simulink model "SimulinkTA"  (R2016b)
settings: Solver=VariableStepAuto  StartTime=0.0  StopTime=10000  RelTol=1e-3
libraries: simulink x15, sldrtlib x1
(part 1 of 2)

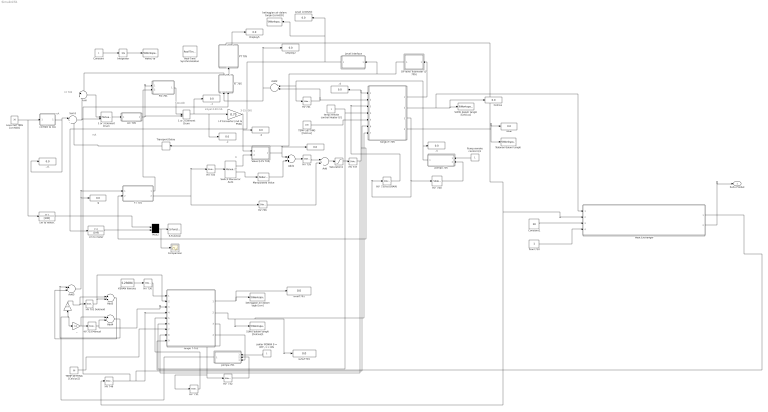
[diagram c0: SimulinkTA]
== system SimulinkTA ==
  note: Cascade
  note: 3-15 PSIG
  note: sinyal 4-20 mA
  note: mA
  note: mA
  note: A
  note: M
  note: LY 705
  ,. : Gain  RequirementInfo={} %GIDa_f98b540b_1780_41dd_a70e_1bad47bc10c1  Gain=1/2
  .{,1..5,9,11} (8 alike) : Display
  .. : Gain  RequirementInfo={} %GIDa_8e0160ac_725a_48f6_95bf_1d56de90cc87  Gain=1/2
  1 or 2 Element Drum : ManualSwitch  RequirementInfo={} %GIDa_50f61c56_16a2_43dc_89b1_2e4d65b653a3  CurrentSetting=0
  1 or 3 Element Drum : ManualSwitch  RequirementInfo={} %GIDa_52ca6b7f_6063_4425_9fdd_553e1b81c659  CurrentSetting=0
  Add : Sum  RequirementInfo={} %GIDa_33aeec0d_9e6c_469e_a3ee_407601759ac2
  Add1 : Sum  RequirementInfo={} %GIDa_8e166b0c_1a9c_4ce2_9319_8c6bd7aad9d2
  Add2 : Sum  RequirementInfo={} %GIDa_713da8c0_9236_4d12_ba44_68ec175b8b10  Inputs=+-
  Add3 : Sum  RequirementInfo={} %GIDa_be23a2ac_e2a6_474d_b9c0_3f98fa9e31fd  Inputs=+-
  Add4 : Sum  RequirementInfo={} %GIDa_40610020_3c23_44b6_97d5_d48497f2e700  Inputs=+-
  Add5 : Sum  RequirementInfo={} %GIDa_806e11a4_cf6f_4655_9173_03499af1af91
  Celcius : Display
  Comparison : Scope
  Constant : Constant  RequirementInfo={} %GIDa_2e5088a9_5b13_476f_95c2_5b910ea94592
  Constant1 : Constant  Value=28
  DP level Trasmitter (LT 705) : Subsystem  RequirementInfo={} %GIDa_91b3a82a_3a49_4232_a21b_3a53aa669424
  Display2 : Display
  Display5 : Display
  FIC 701 : Subsystem  RequirementInfo={} %GIDa_a8cdff3a_9de8_4317_845b_7d10f14f6ae7
  FT 701 : Subsystem  RequirementInfo={} %GIDa_7c1594a4_5410_4ceb_b93e_be43770988d4
  FT 705 : Subsystem  RequirementInfo={} %GIDa_b73ffb92_9bd8_4e1a_9659_5756a25f0d2c
  "HV  731 " : simulink/Math Operations/Slider Gain  low=0  gain=0  high=1
  HV  732 : simulink/Math Operations/Slider Gain  low=0  gain=0  high=1
  "HV  739 to DRAIN " : simulink/Math Operations/Slider Gain  low=0  gain=0  high=1
  "HV  740 " : simulink/Math Operations/Slider Gain  low=0  gain=0  high=1
  HV 701 Selenoid : simulink/Math Operations/Slider Gain  low=0  gain=0  high=1
  HV 730 : simulink/Math Operations/Slider Gain  low=0  gain=0  high=1
  HV 733 Manual : simulink/Math Operations/Slider Gain  low=0  gain=0  high=1
  "HV 734 " : simulink/Math Operations/Slider Gain  low=0  gain=1  high=1
  HV 735 : simulink/Math Operations/Slider Gain  low=0  gain=1  high=1
  "HV 736 " : simulink/Math Operations/Slider Gain  low=0  gain=0  high=1
  "HV 737 " : simulink/Math Operations/Slider Gain  low=0  gain=1  high=1
  "HV 741 " : simulink/Math Operations/Slider Gain  low=0  gain=0  high=1
  HV 746 : simulink/Math Operations/Slider Gain  low=0  gain=0  high=1
  Heat Exchanger : Subsystem
  I-P Converter (mA to PSIG) : Gain  RequirementInfo={} %GIDa_f426d195_d862_463c_9f94_379edd20df78  Gain=0.75
  Integrator : Integrator  RequirementInfo={} %GIDa_73503aa6_2a92_4f4f_9bc4_a531c9719bd6
  KERAN liter/sec : Constant  RequirementInfo={} %GIDa_919a1f09_4405_4c75_a137_f373f18aebd0  Value=0.23084
  LIC 705 : Subsystem  RequirementInfo={} %GIDa_369aca42_e7c0_40f4_8e28_9a6ab2f6df2e
  Level (cmH2O) : Display
  Level SETTING [cmH2O] : Constant  RequirementInfo={} %GIDa_b606e8a9_0597_4d4e_9a3c_ddc012e3713e  Value=20
  Level interface : Subsystem
  Manipulated Value : simulink/Math Operations/Slider Gain  low=0  gain=0  high=1
  Mux2 : Mux  RequirementInfo={} %GIDa_536e6ffc_08cb_4607_84dd_83a51ca6239a  Inputs=2
  PT 705 : Subsystem  RequirementInfo={} %GIDa_f840a07e_6e94_42a6_b25a_e5c048ff3908
  Pump remote control 0/1 : Constant  RequirementInfo={} %GIDa_607b4290_daa3_4be3_9ffe_c29a85919171
  Real-Time Synchronization : sldrtlib/Real-Time Synchronization  SampleTime=0.1  MaxMissedTicks=10  ShowMissedTicks=off  YieldWhenWaiting=off
  S-Function : S-Function  RequirementInfo={} %GIDa_0650cf3a_5639_43d4_998f_7c01600198ab  FunctionName=animtank  Parameters=1  SFunctionDeploymentMode=off  EnableBusSupport=off
  SUHU dalam tangki [Celcius] : ToWorkspace  VariableName=suhu  SampleTime=-1
  SUHU dalam tangki [Celcius]1 : ToWorkspace  VariableName=suhuT701  SampleTime=-1
  Saturation1 : Saturate  RequirementInfo={} %GIDa_cd8c3b9f_0cdd_4174_bcfc_9050506be7ec  UpperLimit=1  LowerLimit=-999999999999999999999999999999999999999999999999999999
  Sum : Sum  RequirementInfo={} %GIDa_f21b71bf_1a6a_4553_b306_4403267bbf57
  Sum1 : Sum  RequirementInfo={} %GIDa_6a427bec_d8ce_4fbe_8754_7b0e1e058e02  Inputs=|+-
  Switch Manual or Auto : simulink/Signal Routing/Manual Variant Sink  NumChoices=2  OverrideUsingVariant=V_1
  TEMP SETTING [Celcius] : Constant  RequirementInfo={} %GIDa_a0082f11_e175_4a79_988b_b8058d6537c5  Value=100
  TEMP SETTING [Celcius]1 : Constant  RequirementInfo={} %GIDa_0bffe608_b418_4e2c_881b_b7b7f3d02c07  Value=58
  "Tekanan dalam tangki " : ToWorkspace  VariableName=Pressure  SampleTime=-1
  Transport Delay : TransportDelay
  Valve (LCV 705) : Subsystem  RequirementInfo={} %GIDa_3844e563_c3df_4c65_8da6_3de284a6d4c1
  cm to meter : TransferFcn  RequirementInfo={} %GIDa_f0868251_1793_40cd_a53d_527cb2fa9c42  Denominator=[100]
  cm to meter. : TransferFcn  RequirementInfo={} %GIDa_1b575afd_8e8e_4baf_a484_d97b38fbf8ac  Denominator=[100]
  cmH2O to mA : Subsystem  RequirementInfo={} %GIDa_cc461a43_9965_4ae5_9710_36f1af421479
  flow t710 : Constant
  ketinggian air dalam tagki [cm] : ToWorkspace  VariableName=levelT701  SampleTime=-1
  ketinggian air dalam tangki [cmH2O] : ToWorkspace  VariableName=level  SampleTime=-1
  levelT701 : Display
  mbar : Display
  pompa 701 : Subsystem  RequirementInfo={} %GIDa_9039f252_afba_432d_871e_a333ebf612b1
  pompa 705 : Subsystem  RequirementInfo={} %GIDa_a2156736_65ee_43f0_a76e_3439dd7fe0a0
  "saklar POMPA 0 = OFF, 1 = ON" : Constant  RequirementInfo={} %GIDa_6e029c51_d003_4219_97b6_ff91aedd926b
  suhuT701 : Display
  tangki F-705 : Subsystem  RequirementInfo={} %GIDa_ce866985_5924_40b0_9c43_161a26f9d3fc
  tangki T-701 : Subsystem  RequirementInfo={} %GIDa_c1bbe68a_d7d3_439e_ab0d_2ecc6b9f0754
  temp remote control Heater 0/1 : Constant  RequirementInfo={} %GIDa_f198997b_9acc_483d_843c_45cb6b1aec35
  waktu-ta' : ToWorkspace  VariableName=time  SampleTime=-1
  Suhu Produk : Outport
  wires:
  Constant/1 -> Integrator/1
  tangki F-705/3(flow out [Liter/sec]) -> "HV  740 "/1, "HV  739 to DRAIN "/1
  "HV  739 to DRAIN "/1 -> tangki F-705/3(In6)
  "HV 736 "/1 -> Add/2
  HV 735/1 -> Add/1
  Add/1 -> Saturation1/1
  TEMP SETTING [Celcius]/1 -> tangki F-705/5(setting)
  FT 705/1(Out1) -> Sum/1
  Sum/1 -> 1 or 3 Element Drum/1
  FIC 701/1(Control) -> 1 or 2 Element Drum/1
  Saturation1/1 -> "HV 737 "/1
  Mux2/1 -> S-Function/1, Comparison/1
  Pump remote control 0/1/1 -> pompa 705/1(saklar remote)
  Integrator/1 -> waktu-ta'/1
  FT 705/2("Out2 ") -> PT 705/1("In ")
  "HV 741 "/1 -> Add2/2, tangki F-705/2(In2)
  "HV 734 "/1 -> Switch Manual or Auto/1
  Switch Manual or Auto/2 -> Manipulated Value/1
  Manipulated Value/1 -> Add1/2
  Add1/1 -> HV 735/1
  FT 701/2(Out2) -> "HV 734 "/1, "HV 736 "/1
  FT 701/1(Out1) -> FIC 701/2(flow in)
  Add2/1 -> FT 705/1(In), Display2/1
  pompa 705/1(Out1) -> .5/1, Add2/1, "HV 741 "/1
  tangki F-705/4(Pressure (Pa)) -> "Tekanan dalam tangki "/1, mbar/1
  cm to meter/1 -> Mux2/2
  cm to meter./1 -> Mux2/1
  Level SETTING [cmH2O]/1 -> cmH2O to mA/1(In1), cm to meter./1
  cmH2O to mA/1(Out1) -> .11/1, Sum1/1
  Switch Manual or Auto/1 -> Valve (LCV 705)/2(In2)
  I-P Converter (mA to PSIG)/1 -> Valve (LCV 705)/1(In1), .3/1
  Valve (LCV 705)/1(Out1) -> ./1, Add1/1
  1 or 2 Element Drum/1 -> .2/1, I-P Converter (mA to PSIG)/1, .1/1
  Sum1/1 -> Sum/2, 1 or 3 Element Drum/2
  LIC 705/1(Control) -> 1 or 2 Element Drum/2, FIC 701/1(Set Point)
  1 or 3 Element Drum/1 -> LIC 705/1(error)
  tangki T-701/1(level [cm]) -> ketinggian air dalam tagki [cm]/1, levelT701/1
  HV 730/1 -> tangki T-701/1(In1)
  KERAN liter/sec/1 -> HV 730/1
  HV 746/1 -> FT 705/2(Valve), tangki F-705/6(In3), tangki T-701/4(In4)
  pompa 701/1(Out1) -> ,./1, ../1
  "saklar POMPA 0 = OFF, 1 = ON"/1 -> pompa 701/1(saklar remote)
  tangki T-701/3(debit out (Liter/sec)) -> "HV  731 "/1, HV  732/1
  "HV  731 "/1 -> tangki T-701/5(In6)
  temp remote control Heater 0/1/1 -> tangki T-701/6(remote on/off), tangki F-705/4(remote on/off)
  TEMP SETTING [Celcius]1/1 -> tangki T-701/7(setting)
  HV 733 Manual/1 -> tangki T-701/3(In3), Add4/2
  HV 701 Selenoid/1 -> tangki T-701/2(In2), Add3/2
  Add3/1 -> Add5/2
  Add4/1 -> Add5/1
  ../1 -> Add3/1, HV 701 Selenoid/1
  ,./1 -> Add4/1, HV 733 Manual/1
  tangki F-705/1(level [cm]) -> DP level Trasmitter (LT 705)/1(In1)
  DP level Trasmitter (LT 705)/1(Out1) -> Transport Delay/1, Level interface/1(In1)
  Level interface/1(Out1) -> Level (cmH2O)/1, ketinggian air dalam tangki [cmH2O]/1, cm to meter/1
  tangki T-701/4(to pompa) -> pompa 701/3(LSL 701)
  PT 705/2(Pressure Flow) -> Display5/1
  "HV 737 "/1 -> tangki T-701/8(In7), FT 701/2(valve), .4/1, tangki F-705/1(In1)
  HV  732/1 -> pompa 701/2(In2)
  "HV  740 "/1 -> pompa 705/2(In2)
  Add5/1 -> FT 701/1(In), .9/1
  tangki T-701/2(suhu [Celcius]) -> SUHU dalam tangki [Celcius]1/1, tangki F-705/7(Heat dari T-701), suhuT701/1
  Transport Delay/1 -> Sum1/2
  tangki F-705/2(suhu [Celcius]) -> Heat Exchanger/1(In1), Celcius/1, SUHU dalam tangki [Celcius]/1
  PT 705/1(Out1) -> Heat Exchanger/2(In2), HV 746/1
  Constant1/1 -> Heat Exchanger/3(In3)
  flow t710/1 -> Heat Exchanger/4(In4)
  Heat Exchanger/1(Suhu Kondensasi) -> tangki T-701/9(Suhu Heat Exchanger)
  Heat Exchanger/2(Suhu Produk) -> Suhu Produk/1

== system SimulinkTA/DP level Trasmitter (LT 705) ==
  note: mA
  In1 : Inport  RequirementInfo={} %GIDa_1eb3f1c2_5012_4cad_855b_2958c3d38ffb
  Bias : Bias  RequirementInfo={} %GIDa_58e9c4c0_21ff_4a03_84f0_4ce1e2662299  Bias=4
  DP Level Transmitter Transfer Function : TransferFcn  RequirementInfo={} %GIDa_eee34651_116f_407c_b9f8_a46affdd8c9a  Numerator=[0.16]  Denominator=[1 1]
  Saturation : Saturate  RequirementInfo={} %GIDa_ada29e25_1fd3_4206_a0fe_ed11e72ed176  UpperLimit=100  LowerLimit=0
  Out1 : Outport  RequirementInfo={} %GIDa_9d16e56c_2f4e_4061_b9df_babf82f61ec4
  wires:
  Bias/1 -> Out1/1
  In1/1 -> Saturation/1
  Saturation/1 -> DP Level Transmitter Transfer Function/1
  DP Level Transmitter Transfer Function/1 -> Bias/1

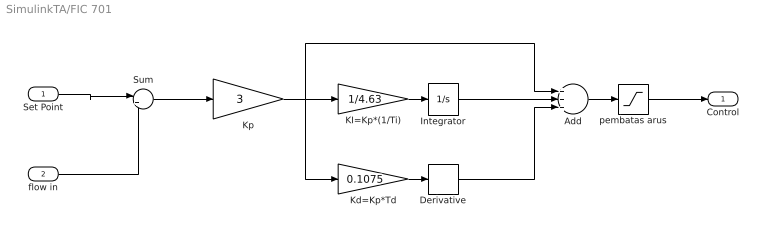
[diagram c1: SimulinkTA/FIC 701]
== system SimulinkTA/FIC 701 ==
  Set Point : Inport  RequirementInfo={} %GIDa_324f346b_80f6_4eeb_baa7_a739d0073a64
  flow in : Inport  RequirementInfo={} %GIDa_5ed90229_9be7_4949_82bd_1c5191f280ea  Port=2
  Add : Sum  RequirementInfo={} %GIDa_15deaa71_a684_46d7_8122_73e07a876b7f  Inputs=+++
  Derivative : Derivative  RequirementInfo={} %GIDa_9c52db40_5651_421e_aa6c_2abf2da229d9
  Integrator : Integrator  RequirementInfo={} %GIDa_8ed4c423_4cc0_4b59_be2d_7167c1b33641  WrappedStateUpperValue=1  WrappedStateLowerValue=0  AbsoluteTolerance=0.000001
  KI=Kp*(1/Ti) : Gain  RequirementInfo={} %GIDa_e0e428a7_39aa_4d35_9287_129381d2bdb6  Gain=1/4.63
  Kd=Kp*Td : Gain  RequirementInfo={} %GIDa_a8fec24f_458c_4778_9ae6_6eb8972fcc58  Gain=0.1075
  Kp : Gain  RequirementInfo={} %GIDa_8e1a382b_fde3_48e4_892d_3c7ebd8edd9a  Gain=3
  Sum : Sum  RequirementInfo={} %GIDa_246cbfd3_5e28_4028_b105_e3101a24dce3  Inputs=|+-
  pembatas arus : Saturate  RequirementInfo={} %GIDa_8de01058_7f9d_485c_90b3_6907439db83d  UpperLimit=20  LowerLimit=4  LinearizeAsGain=off  ZeroCross=off
  Control : Outport  RequirementInfo={} %GIDa_4b2e259f_2bc4_4e50_9d25_d227638a7e45
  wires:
  pembatas arus/1 -> Control/1
  Set Point/1 -> Sum/1
  Derivative/1 -> Add/3
  Kd=Kp*Td/1 -> Derivative/1
  KI=Kp*(1/Ti)/1 -> Integrator/1
  Integrator/1 -> Add/2
  Sum/1 -> Kp/1
  Kp/1 -> Add/1, KI=Kp*(1/Ti)/1, Kd=Kp*Td/1
  flow in/1 -> Sum/2
  Add/1 -> pembatas arus/1

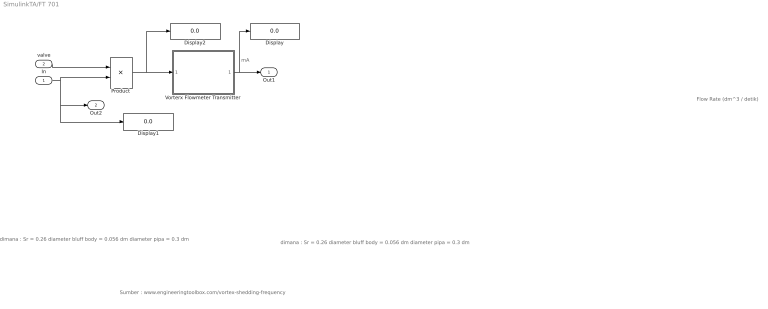
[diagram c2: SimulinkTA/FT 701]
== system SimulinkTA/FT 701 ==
  note: dimana : Sr = 0.26 diameter bluff body = 0.056 dm diameter pipa = 0.3 dm
  note: Sumber : www.engineeringtoolbox.com/vortex-shedding-frequency
  note: mA
  note: dimana : Sr = 0.26 diameter bluff body = 0.056 dm diameter pipa = 0.3 dm
  note: Flow Rate (dm^3 / detik)
  In : Inport  RequirementInfo={} %GIDa_b8d848c2_2911_47dc_96b8_30bc6067c079
  valve : Inport  RequirementInfo={} %GIDa_c0e35d82_3a45_4c27_8ff2_a1822ceec22b  Port=2
  Display : Display
  Display1 : Display
  Display2 : Display
  Product : Product  RequirementInfo={} %GIDa_595abe10_ac01_44d9_bc50_37596a372820
  Vorterx Flowmeter Transmitter : Subsystem  RequirementInfo={} %GIDa_c3a464df_94d7_42b7_baee_52d014caaae7
  Out1 : Outport  RequirementInfo={} %GIDa_1cf06766_2529_43d4_99e4_8bd828d323fc
  Out2 : Outport  RequirementInfo={} %GIDa_6f056275_4462_4c57_ac99_2a76f3dcdf0e  Port=2
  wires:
  valve/1 -> Product/1
  In/1 -> Display1/1, Out2/1, Product/2
  Vorterx Flowmeter Transmitter/1(Out1) -> Out1/1, Display/1
  Product/1 -> Display2/1, Vorterx Flowmeter Transmitter/1(In1)

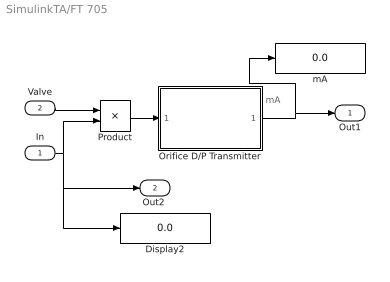
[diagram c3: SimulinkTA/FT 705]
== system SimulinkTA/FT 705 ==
  note: mA
  In : Inport  RequirementInfo={} %GIDa_f3c7ff77_d86d_4eb5_84c4_1f3baeebc0aa
  Valve : Inport  RequirementInfo={} %GIDa_eef1c914_c385_47be_acc7_ebc407a52e57  Port=2
  Display2 : Display
  Orifice D/P Transmitter : Subsystem  RequirementInfo={} %GIDa_f9f38d8f_ec91_4141_85ce_4e8fc10cd6a1
  Product : Product
  mA : Display
  Out1 : Outport  RequirementInfo={} %GIDa_04c1a58a_c817_4ad6_a918_7ac37ecd04d6
  "Out2 " : Outport  RequirementInfo={} %GIDa_6ccc8379_ec08_4508_bb2e_d09c5228564c  Port=2
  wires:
  In/1 -> Product/2, Display2/1, "Out2 "/1
  Orifice D/P Transmitter/1(Out1) -> mA/1, Out1/1
  Valve/1 -> Product/1
  Product/1 -> Orifice D/P Transmitter/1(In1)

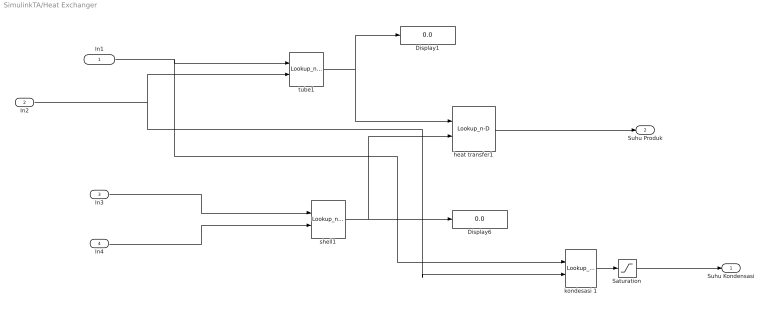
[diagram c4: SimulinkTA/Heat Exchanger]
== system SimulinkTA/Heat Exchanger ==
  In1 : Inport
  In2 : Inport  Port=2
  In3 : Inport  Port=3
  In4 : Inport  Port=4
  Display1 : Display
  Display6 : Display
  Saturation : Saturate  UpperLimit=5
  heat transfer1 : Lookup_n-D  BreakpointsForDimension1=[20,25,30]  BreakpointsForDimension2=[22,23,28,32,34,36,38,39,40,41,42,43,44,45,46,47,48,49,50,51,52,53,54,55,56,57,58,59,60,61,62]  Table=reshape([28,30,33,29,31,34,29,31,34,30,32,35,31,33,36,31,34,36,31,34,37,32,34,38,32,35,39,33,35,40,33,36,40,34,36,41,35,37,41,35,37,42,36,38,43,37,38,44,37,39,45,37,39,45,38,40,45,38,40,46,38,41,47,38,41,48,38,42,49,38,42,50,38,43,50,39,43,51,39,44,52,39,44,52,39,45,53,39,46,54,39,47,55],3,31)  InternalRulePriority=Speed  RndMeth=Simplest
  kondesasi 1 : Lookup_n-D  BreakpointsForDimension1=[37.7,38.1,38.2,38.4,38.5,38.6,38.7,38.9,40,40.1,40.2,40.3,40.4,40.5,40.6,40.7,40.8,40.9,41,41.1,41.2,41.3,41.4,41.5,41.6,41.7,41.8,41.9,42,42.1,42.2,42.3,42.4,42.5,42.6,42.7,42.8]  BreakpointsForDimension2=[21,22,27,28,32,34,35,37,38,39,40,41,42,43,45,46,48,49,50,51,52,53,54,55,56,57,58,59,60,61,62,63,64,65,66,67,68]  Table=reshape([28,0,0,0,0,0,0,0,0,0,0,0,0,0,0,0,0,0,0,0,0,0,0,0,0,0,0,0,0,0,0,0,0,0,0,0,0,0,28,0,0,0,0,0,0,0,0,0,0,0,0,0,0,0,0,0,0,0,0,0,0,0,0,0,0,0,0,0,0,0,0,0,0,0,0,0,28,0,0,0,0,0,0,0,0,0,0,0,0,0,0,0,0,0,0,0,0,0,0,0,0,0,0,0,0,0,0,0,0,0,0,0,0,0,28,0,0,0,0,0,0,0,0,0,0,0,0,0,0,0,0,0,0,0,0,0,0,0,0,0,0,0,0,0,0,0,0,0,0,0,0,0,28,0,0,0,0,0,0,0,0,0,0,0,0,0,0,0,0,0,0,0,0,0,0,0,0,0,0,0,0,0,0,0,0,0,0,0,0,0,28,0,0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  InternalRulePriority=Speed  RndMeth=Simplest
  shell1 : Lookup_n-D  BreakpointsForDimension1=[22,23,24,25,26,27,28,29,30,31,32,33,34,35,36,37,38,39,40,41,42,43,44,45,46,47,48,49,50,51]  BreakpointsForDimension2=[20,30,40]  Table=reshape([20,20,20,20,20,20,20,20,20,20,20,20,20,20,20,20,20,20,20,20,20,20,20,20,20,20,20,20,20,20,30,30,30,30,30,30,30,30,30,30,30,30,30,30,30,30,30,30,30,30,30,30,30,30,30,30,30,30,30,30,40,40,40,40,40,40,40,40,40,40,40,40,40,40,40,40,40,40,40,40,40,40,40,40,40,40,40,40,40,40],30,3)  InternalRulePriority=Speed  RndMeth=Simplest
  tube1 : Lookup_n-D  BreakpointsForDimension1=[37.7,38.2,38.6,39.1,39.6,40,40.2,40.4,40.9,41,41.1,41.2,41.3,41.4,41.5,41.6,41.7,41.8]  BreakpointsForDimension2=[50.5,60.5,65.5]  Table=reshape([20,20,24,24,25,26,26,27,28,29,29,30,31,32,32,33,34,34,21,23,23,23,25,26,28,29,29,30,31,33,35,35,35,36,36,37,22,28,28,32,34,36,38,39,39,40,41,43,44,45,46,47,48,48],18,3)  InternalRulePriority=Speed  RndMeth=Simplest
  Suhu Kondensasi : Outport
  Suhu Produk : Outport  Port=2
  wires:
  In2/1 -> kondesasi 1/2, tube1/2
  In1/1 -> kondesasi 1/1, tube1/1
  tube1/1 -> Display1/1, heat transfer1/1
  heat transfer1/1 -> Suhu Produk/1
  shell1/1 -> heat transfer1/2, Display6/1
  In4/1 -> shell1/2
  In3/1 -> shell1/1
  kondesasi 1/1 -> Saturation/1
  Saturation/1 -> Suhu Kondensasi/1

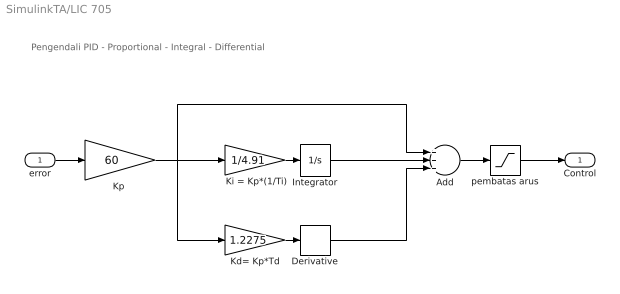
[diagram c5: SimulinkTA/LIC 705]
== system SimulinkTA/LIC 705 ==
  note: Pengendali PID - Proportional - Integral - Differential
  error : Inport  RequirementInfo={} %GIDa_dd45f130_5e06_4a08_96d6_82784c8b669b
  " Ki = Kp*(1/Ti)" : Gain  RequirementInfo={} %GIDa_346b1e91_1c59_43a3_9052_7741d6bb7140  Gain=1/4.91
  Add : Sum  RequirementInfo={} %GIDa_71aef157_9422_4e61_9508_acd0b7c5c00a  Inputs=+++
  Derivative : Derivative  RequirementInfo={} %GIDa_29cba799_ea93_4ef6_8db0_e83d8d126ea8
  Integrator : Integrator  RequirementInfo={} %GIDa_6717b320_0546_4ca8_a8d5_c68c50b6bacd  WrappedStateUpperValue=1  WrappedStateLowerValue=0  AbsoluteTolerance=0.000001
  Kd= Kp*Td : Gain  RequirementInfo={} %GIDa_d15db0ae_a410_43fa_87d6_0f4128930a65  Gain=1.2275
  "Kp " : Gain  RequirementInfo={} %GIDa_ef8245be_e217_43e9_a890_e3f1d4b98027  Gain=60
  pembatas arus : Saturate  RequirementInfo={} %GIDa_655a4809_8b2d_4a76_85d9_c787e0a18bf5  UpperLimit=20  LowerLimit=4  LinearizeAsGain=off  ZeroCross=off
  Control : Outport  RequirementInfo={} %GIDa_693e0adf_1111_48a6_bc02_1f4e93b86194
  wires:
  Derivative/1 -> Add/3
  Kd= Kp*Td/1 -> Derivative/1
  " Ki = Kp*(1/Ti)"/1 -> Integrator/1
  Integrator/1 -> Add/2
  error/1 -> "Kp "/1
  "Kp "/1 -> Add/1, " Ki = Kp*(1/Ti)"/1, Kd= Kp*Td/1
  Add/1 -> pembatas arus/1
  pembatas arus/1 -> Control/1

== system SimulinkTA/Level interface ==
  In1 : Inport
  Bias : Bias  RequirementInfo={} %GIDa_c531b1b5_886c_4ac8_8623_3d6c8e6dde79  Bias=-4
  Transfer Fcn : TransferFcn  Denominator=[0.16]
  Out1 : Outport
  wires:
  In1/1 -> Bias/1
  Transfer Fcn/1 -> Out1/1
  Bias/1 -> Transfer Fcn/1

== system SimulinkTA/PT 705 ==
  note: L/s
  note: mA
  "In " : Inport  RequirementInfo={} %GIDa_e9a98173_53e5_4ac0_b43d_5cbb92f3ad80
  Bias : Bias  RequirementInfo={} %GIDa_4eca5bbc_333a_41d1_ae81_664ae3dadbcb  Bias=4
  Display : Display
  "Pressure Transmitter " : TransferFcn  RequirementInfo={} %GIDa_0520f988_442d_4c53_a742_91df10ecb3ff  Numerator=[16]  Denominator=[3 1]
  pressure interface : Lookup_n-D  NumberOfTableDimensions=1  BreakpointsForDimension1=[4,5,6,7,8,9,10,11,12,13,14,15,16,17,18,19,20]  Table=[0,1.875,3.75,5.625,7.5,9.375,11.25,13.125,15,16.875,18.75,20.625,22.5,24.375,26.25,28.125,30]  InternalRulePriority=Speed  RndMeth=Simplest
  Out1 : Outport  RequirementInfo={} %GIDa_90610641_c374_48be_a99d_cce7686848a9
  Pressure Flow : Outport  RequirementInfo={} %GIDa_0f23660a_b278_4b6f_8674_e20e74fc8a0c  Port=2
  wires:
  "Pressure Transmitter "/1 -> Bias/1
  "In "/1 -> "Pressure Transmitter "/1, Out1/1
  Bias/1 -> pressure interface/1
  pressure interface/1 -> Pressure Flow/1, Display/1

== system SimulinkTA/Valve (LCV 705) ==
  In1 : Inport  RequirementInfo={} %GIDa_071fb54c_b27d_4ca7_965d_47a1c0c6af2b
  In2 : Inport  RequirementInfo={} %GIDa_990ad555_466a_459a_861f_7c0da9c5df6a  Port=2
  Display1 : Display
  Display2 : Display
  Display3 : Display
  Product : Product  RequirementInfo={} %GIDa_286bcfab_fb18_430a_b2ef_fe181dd3aa79
  Tekanan ke posisi katup : Lookup_n-D  RequirementInfo={} %GIDa_66e685fd_b6da_4f9a_878e_acd133167906  NumberOfTableDimensions=1  BreakpointsForDimension1=single([3,4,5,6,7,8,9,10,11,12,13,14,15]);  Table=single([0,0.08333333,0.16666666,0.25,0.33333333,0.41666666,0.5,0.58333333,0.66666666,0.75,0.83333333,0.91666666,1]);  InternalRulePriority=Speed  RndMeth=Simplest
  Out1 : Outport  RequirementInfo={} %GIDa_0d5828b4_d70f_41ad_89e5_3850f8cab4eb
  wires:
  In2/1 -> Display1/1, Product/2
  Product/1 -> Out1/1
  In1/1 -> Display3/1, Display2/1, Tekanan ke posisi katup/1
  Tekanan ke posisi katup/1 -> Product/1

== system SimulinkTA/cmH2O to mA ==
  note: mA
  In1 : Inport  RequirementInfo={} %GIDa_4abbce3a_4ace_4b20_bf02_e2879ea46cbc
  Bias : Bias  RequirementInfo={} %GIDa_cdc4bca7_a50e_40d2_b714_2300d9311ba2  Bias=4
  Gain : Gain  RequirementInfo={} %GIDa_46d57766_a1a0_4448_a107_d208a92ded48  Gain=0.16
  Out1 : Outport  RequirementInfo={} %GIDa_8f484192_46e3_4c72_8ac4_1fec9aee939e
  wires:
  In1/1 -> Gain/1
  Gain/1 -> Bias/1
  Bias/1 -> Out1/1

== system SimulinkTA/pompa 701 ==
  saklar remote : Inport  RequirementInfo={} %GIDa_f0dbef85_ccf0_43aa_8a71_7b6447f6615c
  In2 : Inport  RequirementInfo={} %GIDa_4002fada_6885_4b1c_9113_1802846a976e  Port=2
  LSL 701 : Inport  RequirementInfo={} %GIDa_3faa94ff_f290_4932_83e8_eb9e39ea2cf9  Port=3
  Kapasitas Maksimum Pompa 60 LPM : Saturate  RequirementInfo={} %GIDa_0c0476b5_fefd_405a_a481_b82eb14eae8a  UpperLimit=1  LowerLimit=-999999999999999999999999999999999999999999
  Product1 : Product  RequirementInfo={} %GIDa_a7db1029_012f_45bb_bcf1_9f8c3aae344f  Inputs=3
  Out1 : Outport  RequirementInfo={} %GIDa_2399ff75_e557_47f9_8598_6094e5d9d0ec
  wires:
  Kapasitas Maksimum Pompa 60 LPM/1 -> Out1/1
  Product1/1 -> Kapasitas Maksimum Pompa 60 LPM/1
  LSL 701/1 -> Product1/3
  In2/1 -> Product1/2
  saklar remote/1 -> Product1/1

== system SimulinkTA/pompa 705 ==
  saklar remote : Inport  RequirementInfo={} %GIDa_ce4c0bdc_02a0_4e15_a756_ca46c67d0d4a
  In2 : Inport  RequirementInfo={} %GIDa_c55bffd7_d080_40f3_8a65_61f58044dd3b  Port=2
  Kapasitas Maksimum Pompa 60 LPM : Saturate  RequirementInfo={} %GIDa_56428f8a_5c44_4c2d_a464_266cd883adae  UpperLimit=1  LowerLimit=-9999999999999999999999999999999999999999
  Product : Product  RequirementInfo={} %GIDa_b667c3b9_3fc5_4471_afd4_311206029d39
  To Workspace : ToWorkspace  VariableName=flow_out  SampleTime=-1
  Out1 : Outport  RequirementInfo={} %GIDa_7c185da8_fffc_40e3_a89c_492e4dadb701
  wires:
  Product/1 -> Kapasitas Maksimum Pompa 60 LPM/1
  In2/1 -> Product/2
  saklar remote/1 -> Product/1
  Kapasitas Maksimum Pompa 60 LPM/1 -> To Workspace/1, Out1/1

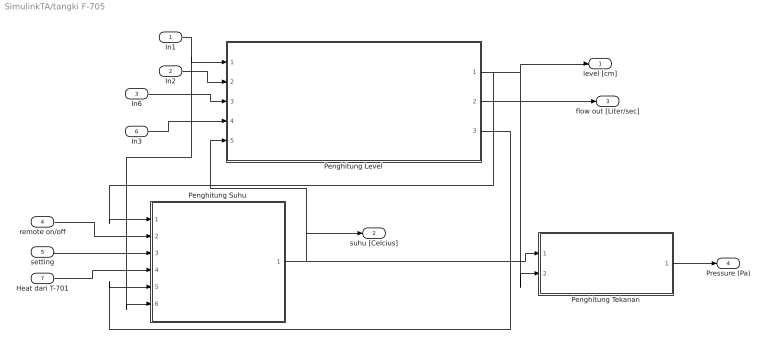
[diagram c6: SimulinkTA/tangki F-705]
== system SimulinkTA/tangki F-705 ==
  In1 : Inport  RequirementInfo={} %GIDa_6b8bd25f_91e1_4a1b_a63a_470dd857bdf8
  In2 : Inport  RequirementInfo={} %GIDa_b4f5d8fe_81c1_4e70_ba2a_042fbdb8f207  Port=2
  In6 : Inport  RequirementInfo={} %GIDa_f921b76f_10f0_46da_83e1_b6c1e41acc84  Port=3
  remote on/off : Inport  RequirementInfo={} %GIDa_440d5800_6004_4907_9105_aa6246f6e84c  Port=4
  setting : Inport  RequirementInfo={} %GIDa_3a574657_fc19_4d06_a2da_9b74b94f6da3  Port=5
  In3 : Inport  RequirementInfo={} %GIDa_57198f3d_1064_4541_9626_ea9352dddd9b  Port=6
  Heat dari T-701 : Inport  RequirementInfo={} %GIDa_2308a404_2f63_4792_902e_8b07c82c1311  Port=7
  Penghitung Level : Subsystem  RequirementInfo={} %GIDa_03a45ce1_963a_49c8_8893_4047c5627c16
  Penghitung Suhu : Subsystem  RequirementInfo={} %GIDa_2bb4627e_45b1_4c10_930e_f7c7a01facba
  Penghitung Tekanan : Subsystem  RequirementInfo={} %GIDa_e3e8e49b_8a10_4d58_b177_60e5d5553077
  level [cm] : Outport  RequirementInfo={} %GIDa_f9324d2d_4619_4288_8a58_a636f2d48ecb
  suhu [Celcius] : Outport  RequirementInfo={} %GIDa_3a96dc9d_4bc0_45bb_ad65_b60b3553aafa  Port=2
  flow out [Liter/sec] : Outport  RequirementInfo={} %GIDa_2267fa52_2237_49a5_b68a_c6fb6a9cbb87  Port=3
  Pressure (Pa) : Outport  RequirementInfo={} %GIDa_da2f54a2_04db_4470_a5be_ed715caf9a76  Port=4
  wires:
  Penghitung Suhu/1(suhu) -> suhu [Celcius]/1, Penghitung Level/5(Suhu), Penghitung Tekanan/1(Suhu)
  In2/1 -> Penghitung Level/2(Dari Pompa lewat HV-741)
  In6/1 -> Penghitung Level/3(Drain)
  Penghitung Level/1(level [cmH2O]) -> level [cm]/1, Penghitung Tekanan/2(Level), Penghitung Suhu/1(level[cm])
  remote on/off/1 -> Penghitung Suhu/2(Remote Heater)
  In1/1 -> Penghitung Suhu/6("liter/s T-701 "), Penghitung Level/1(dari T-701)
  Heat dari T-701/1 -> Penghitung Suhu/4(dari Heat T-701)
  In3/1 -> Penghitung Level/4(Pompa 705)
  Penghitung Level/2(debit out (Liter/sec)) -> flow out [Liter/sec]/1
  setting/1 -> Penghitung Suhu/3(Set Point)
  Penghitung Level/3(Liter (Kg)) -> Penghitung Suhu/5(liter(dm^3))
  Penghitung Tekanan/1(Pressure tangki (mbar)) -> Pressure (Pa)/1

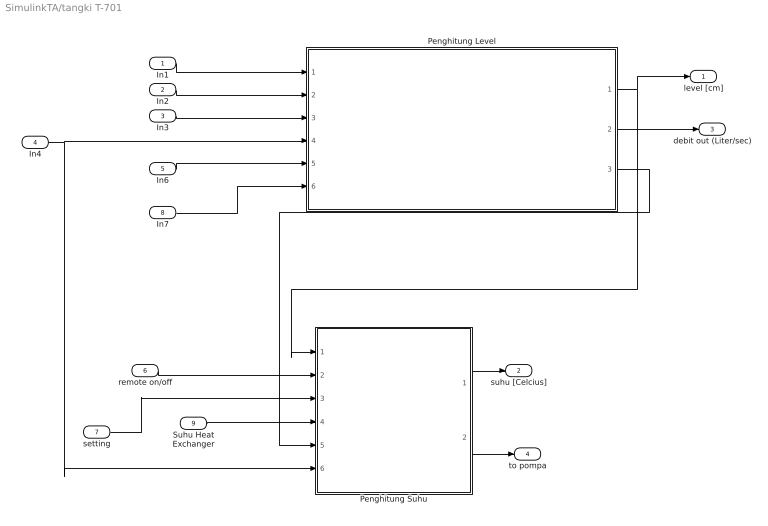
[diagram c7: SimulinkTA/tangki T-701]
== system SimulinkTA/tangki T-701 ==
  In1 : Inport  RequirementInfo={} %GIDa_bcb889f0_8e14_4033_871c_08fd8969ab03
  In2 : Inport  RequirementInfo={} %GIDa_182dc3be_89ad_4058_9f21_8fbcc66bb56d  Port=2
  In3 : Inport  RequirementInfo={} %GIDa_4fe6d71c_85d1_4816_a64f_bad63feab677  Port=3
  In4 : Inport  RequirementInfo={} %GIDa_1bd2da6d_cbd2_4095_9cdb_04f46d418e56  Port=4
  In6 : Inport  RequirementInfo={} %GIDa_3d7e217c_92d7_4a97_9adc_77279aba335d  Port=5
  remote on/off : Inport  RequirementInfo={} %GIDa_180fb63d_11ea_43c5_9d6e_1f37aa0e8a1f  Port=6
  setting : Inport  RequirementInfo={} %GIDa_c1d30b33_d94a_4876_bff4_8ac9b70c51b1  Port=7
  In7 : Inport  RequirementInfo={} %GIDa_004e60c7_1b88_44bf_ba89_5a05d0cf6a13  Port=8
  Suhu Heat Exchanger : Inport  RequirementInfo={} %GIDa_40294428_f7b3_4763_a02a_6a0b6f2ef813  Port=9
  Penghitung Level : Subsystem  RequirementInfo={} %GIDa_6aec6efc_d3f4_4528_aedf_699bf01515c3
  Penghitung Suhu : Subsystem  RequirementInfo={} %GIDa_e0e24de6_f2f7_4a8d_b447_02ea320e5105
  level [cm] : Outport  RequirementInfo={} %GIDa_65216955_8658_4409_8ee1_f3a2b667f001
  suhu [Celcius] : Outport  RequirementInfo={} %GIDa_043b60a9_bf62_4bab_a8fa_8e2919f55607  Port=2
  debit out (Liter/sec) : Outport  RequirementInfo={} %GIDa_f5ac2eab_8593_4570_847d_99dac1fef13d  Port=3
  to pompa : Outport  RequirementInfo={} %GIDa_bc6d46d5_257e_4887_8d6d_6164ec2610eb  Port=4
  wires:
  In1/1 -> Penghitung Level/1(dari keran via HV-730)
  In2/1 -> Penghitung Level/2(Dari Pompa lewat HV-701)
  In3/1 -> Penghitung Level/3(Dari Pompa lewat HV-733)
  In6/1 -> Penghitung Level/5(Drain)
  In7/1 -> Penghitung Level/6(HV 732 ke Pompa)
  Penghitung Level/2(debit out (Liter/sec)) -> debit out (Liter/sec)/1
  Penghitung Level/1(level [cm]) -> Penghitung Suhu/1(level[cm]), level [cm]/1
  Penghitung Suhu/1(suhu) -> suhu [Celcius]/1
  remote on/off/1 -> Penghitung Suhu/2(Remote Heater)
  Suhu Heat Exchanger/1 -> Penghitung Suhu/4(dari Heat dari kondensasi)
  In4/1 -> Penghitung Suhu/6("liter/s Heat Exchanger "), Penghitung Level/4(Dari Heat-Exc  lewat HV-746)
  setting/1 -> Penghitung Suhu/3(Set Point)
  Penghitung Level/3(Liter (dm^3)) -> Penghitung Suhu/5(liter(dm^3))
  Penghitung Suhu/2(to pompa) -> to pompa/1

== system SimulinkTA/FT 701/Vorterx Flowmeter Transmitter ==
  note: mA
  In1 : Inport  RequirementInfo={} %GIDa_3c82c1d3_80d3_4c55_bed4_e80e32ede62a
  Bias : Bias  RequirementInfo={} %GIDa_43cd0c8e_b2d6_4de3_9e07_dc3ebdbc8b54  Bias=4
  Vortex Flowmeter Transmitter Transfer Function : TransferFcn  RequirementInfo={} %GIDa_0b5c6d43_49ee_4a6b_871a_887aab7c0c28  Numerator=[16]  Denominator=[5 1]
  Out1 : Outport  RequirementInfo={} %GIDa_7237a98e_80bf_4470_b5fb_0b30382425cd
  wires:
  Vortex Flowmeter Transmitter Transfer Function/1 -> Bias/1
  Bias/1 -> Out1/1
  In1/1 -> Vortex Flowmeter Transmitter Transfer Function/1

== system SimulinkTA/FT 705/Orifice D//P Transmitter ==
  In1 : Inport  RequirementInfo={} %GIDa_18e6fd19_ce87_47e3_a6c5_b39e9156739d
  Bias : Bias  RequirementInfo={} %GIDa_b15dcac3_3498_4495_9652_8a3456c23d0d  Bias=4
  Orifice DP Flowmeter Transmitter Transfer Function : TransferFcn  RequirementInfo={} %GIDa_0891602a_0713_4f2a_9e7c_5eaa9802afcb  Numerator=[16]  Denominator=[2 1]
  Out1 : Outport  RequirementInfo={} %GIDa_819e8008_bbf4_4863_95c4_785a31089bed
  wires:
  Bias/1 -> Out1/1
  Orifice DP Flowmeter Transmitter Transfer Function/1 -> Bias/1
  In1/1 -> Orifice DP Flowmeter Transmitter Transfer Function/1

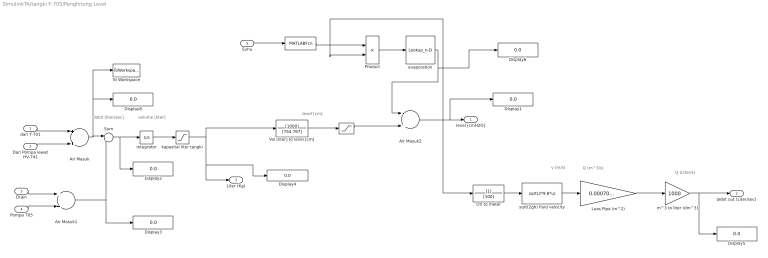
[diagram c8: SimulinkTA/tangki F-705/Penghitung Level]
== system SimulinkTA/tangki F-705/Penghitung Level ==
  note: Q (Liter/s)
  note: Q (m^3/s)
  note: v (m/s)
  note: debit [liter/sec]
  note: level [cm]
  note: volume [liter]
  dari T-701 : Inport  RequirementInfo={} %GIDa_eaae5ac4_e317_46a6_8326_119707a04eb6
  Dari Pompa lewat HV-741 : Inport  RequirementInfo={} %GIDa_f659e66f_f328_49f4_b478_487221b0aa25  Port=2
  Drain : Inport  RequirementInfo={} %GIDa_a4dcbed1_8eaf_4df6_a0c1_c1edcc3eda54  Port=3
  Pompa 705 : Inport  RequirementInfo={} %GIDa_3e0646d3_daea_497c_a7d9_11aac726e74a  Port=4
  Suhu : Inport  RequirementInfo={} %GIDa_5260f4ee_eb02_4a12_96df_c8dafedb793a  Port=5
  " " : MATLABFcn  RequirementInfo="{'linktype_rmi_simulink' 'D' ':376' 'true' 'D/Lamp  (SubSystem)' '' } %GIDa_881f99e2_4b57_4ba8_9c64_fd1139de6537"  MATLABFcn=evaporation
  . : Saturate  RequirementInfo={} %GIDa_c568fbd2_8635_4436_a0cd_fe71f3836946  UpperLimit=119.5  LowerLimit=-999999999999999999999999999999999999999999999999999
  Air Masuk : Sum  RequirementInfo={} %GIDa_40efd31c_6666_44a2_9db1_00799f1a42c7
  Air Masuk1 : Sum  RequirementInfo={} %GIDa_8c93796f_53ce_479d_9c4a_748bcce32f12
  Air Masuk2 : Sum  RequirementInfo={} %GIDa_0565a782_fec0_486c_bd30_3e48483af1c0  Inputs=-+
  Display{1..6,8} (7 alike) : Display
  Integrator : Integrator  RequirementInfo={} %GIDa_bc7e7078_2496_4d2c_ae0d_25b00a8bfd45
  Luas Pipa (m^2) : Gain  RequirementInfo={} %GIDa_36744498_b4b1_4c84_8dfa_412d3c9dadba  Gain=0.000706858347
  Product : Product
  Sum : Sum  RequirementInfo={} %GIDa_bee846a6_7929_4da0_bf8e_fc7d5f4cf6df  Inputs=|+-
  To Workspace : ToWorkspace  VariableName=flow_in  SampleTime=-1
  Vol [liter] to level [cm] : TransferFcn  RequirementInfo={} %GIDa_77aff239_6728_4529_ab73_3a0f291d19be  Numerator=[1000]  Denominator=[754.767]
  cm to meter : TransferFcn  RequirementInfo={} %GIDa_49eebb76_f309_4b8c_849a_173f3160c390  Denominator=[100]
  evaporation : Lookup_n-D  NumberOfTableDimensions=1  BreakpointsForDimension1=[0,20,30,40,50]  Table=[0,0.9,1.1,1.1,1.3]  InternalRulePriority=Speed  RndMeth=Simplest
  kapasital liter tangki : Saturate  RequirementInfo={} %GIDa_32b8a840_b1fb_48f6_8958_bcaddac9c507  UpperLimit=100  LowerLimit=-99999999999999999999999999999999999999999999999999
  m^3 to liter (dm^3) : Gain  RequirementInfo={} %GIDa_4a4d0124_9c77_43dc_b0d6_ca1942f331a8  Gain=1000
  sqrt(2gh) fluid velocity : Fcn  RequirementInfo={} %GIDa_fe0dc4ae_eb31_4760_8e73_3d1402e38ee2  Expr=sqrt(2*9.8*u)
  level [cmH2O] : Outport  RequirementInfo="{'linktype_rmi_simulink' 'D' ':376' 'true' 'D/Lamp  (SubSystem)' '' } %GIDa_eb9b9990_17f3_4907_99f2_531b1ce02cde"
  debit out (Liter/sec) : Outport  RequirementInfo={} %GIDa_6c7017ae_a984_4704_bb94_a5d3bd8d3731  Port=2
  Liter (Kg) : Outport  RequirementInfo={} %GIDa_0857ae42_fc5d_4431_892f_84528d6e9e3f  Port=3
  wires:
  Sum/1 -> Display2/1, Integrator/1
  Air Masuk/1 -> Sum/1, Display8/1, To Workspace/1
  Dari Pompa lewat HV-741/1 -> Air Masuk/2
  dari T-701/1 -> Air Masuk/1
  Integrator/1 -> kapasital liter tangki/1
  Drain/1 -> Air Masuk1/1
  Air Masuk1/1 -> Sum/2, Display3/1
  sqrt(2gh) fluid velocity/1 -> Luas Pipa (m^2)/1
  Luas Pipa (m^2)/1 -> m^3 to liter (dm^3)/1
  Pompa 705/1 -> Air Masuk1/2
  cm to meter/1 -> sqrt(2gh) fluid velocity/1
  kapasital liter tangki/1 -> Vol [liter] to level [cm]/1, Display4/1, Liter (Kg)/1
  Vol [liter] to level [cm]/1 -> ./1
  m^3 to liter (dm^3)/1 -> Display5/1, debit out (Liter/sec)/1
  Product/1 -> evaporation/1
  ./1 -> Air Masuk2/2
  Air Masuk2/1 -> cm to meter/1, Product/2, Display1/1, level [cmH2O]/1
  evaporation/1 -> Display6/1, Air Masuk2/1
  Suhu/1 -> " "/1
  " "/1 -> Product/1

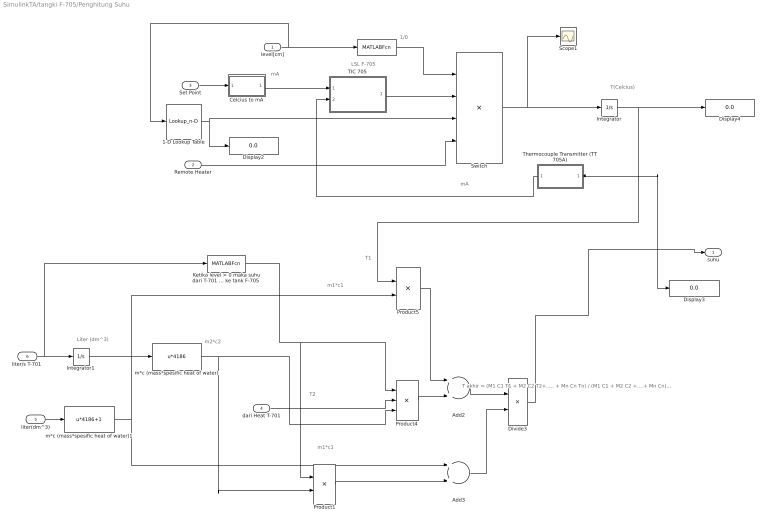
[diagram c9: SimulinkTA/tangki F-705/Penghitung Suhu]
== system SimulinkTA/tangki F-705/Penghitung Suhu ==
  note: mA
  note: mA
  note: T(Celcius)
  note: LSL F-705
  note: 1/0
  note: m1*c1
  note: T1
  note: T2
  note: m2*c2
  note: m1*c1
  note: Liter (dm^3)
  note: T akhir = (M1 C1 T1 + M2 C2 T2+..... + Mn Cn Tn) / (M1 C1 + M2 C2 +....+ Mn Cn) dimana : T akhir = final temperatur M = massa air C = spesific heat (j/Kg C ) T1..n = temperatur subtansi
  level[cm] : Inport  RequirementInfo={} %GIDa_e0b4a970_3d54_4fb0_aff4_8bad3153f225
  Remote Heater : Inport  RequirementInfo={} %GIDa_c65c606e_32ea_4ae9_bbcc_4f8723324b1d  Port=2
  Set Point : Inport  RequirementInfo={} %GIDa_c1afb73a_d3e7_44a7_a71c_a6ebd5a4f030  Port=3
  dari Heat T-701 : Inport  RequirementInfo={} %GIDa_e865df19_7140_4bbd_b654_554030f48665  Port=4
  liter(dm^3) : Inport  RequirementInfo={} %GIDa_d8c17968_031c_448a_870b_c0c002beaf23  Port=5
  "liter/s T-701 " : Inport  RequirementInfo={} %GIDa_1b3527ba_bacc_41d4_854b_bc10a733e129  Port=6
  " " : MATLABFcn  RequirementInfo="{'linktype_rmi_simulink' 'D' ':376' 'true' 'D/Lamp  (SubSystem)' '' } %GIDa_c6ecf6a7_d3cd_4cde_9a8a_d2573dc1e7d7"  MATLABFcn=LSL705
  " Ketika level > 0 maka suhu dari T-701 sudah masuk ke tank F-705" : MATLABFcn  RequirementInfo={} %GIDa_42b6f345_f15e_41dd_919d_842ba00efb6f  MATLABFcn=HeatF705
  1-D Lookup Table : Lookup_n-D  NumberOfTableDimensions=1  BreakpointsForDimension1=[20,30,40,50]  Table=[0.1204,0.08678,0.06899,0.05397]  InternalRulePriority=Speed  RndMeth=Simplest
  Add2 : Sum  RequirementInfo={} %GIDa_9543e41b_2eff_4b16_8586_7709efc37bc1
  Add3 : Sum  RequirementInfo={} %GIDa_d7ff1f8d_9cdd_4cc4_a7ab_6b703f3e1273
  Celcius to mA : Subsystem  RequirementInfo={} %GIDa_92f4a370_4fc3_4d7e_a483_479293201b37
  Display2 : Display
  Display3 : Display
  Display4 : Display
  Divide3 : Product  RequirementInfo={} %GIDa_f54dc0d4_1e03_410c_b725_b27dc9f86047  Inputs=*/
  Integrator : Integrator  RequirementInfo={} %GIDa_6a823ede_e592_4cec_be03_83ab54774d6e  InitialCondition=31.5
  Integrator1 : Integrator  RequirementInfo={} %GIDa_51a86988_38f0_4ae1_981b_8831600f5dbf
  Product1 : Product  RequirementInfo={} %GIDa_ea31269d_8401_4299_a0e1_cf46b0b8a9c4
  Product4 : Product  RequirementInfo={} %GIDa_7dcb86f1_d075_4f60_bb36_9c9743a33213  Inputs=3
  Product5 : Product  RequirementInfo={} %GIDa_e80fb3ad_bdd0_4173_9baa_89108449396c
  Scope1 : Scope
  Switch : Product  RequirementInfo={} %GIDa_3049b312_c1c1_4f55_a749_56ff3d498f77  Inputs=4
  TIC 705 : Subsystem  RequirementInfo={} %GIDa_ae881922_af84_4c5b_acfd_08a0da460abd
  Thermocouple Transmitter (TT 705A) : Subsystem  RequirementInfo={} %GIDa_abf13e74_616c_4b25_9285_b9a37b16b9a9
  m*c (mass*spesific heat of water) : Fcn  RequirementInfo={} %GIDa_aa796e01_e512_4f84_b4e6_ae564545c52e  Expr=u*4186
  m*c (mass*spesific heat of water)1 : Fcn  RequirementInfo={} %GIDa_195e02d6_b07f_4f1e_bea3_4289a702f6f7  Expr=u*4186+1
  suhu : Outport  RequirementInfo={} %GIDa_864eb9f8_2ab7_407b_810a_d791316e6ecd
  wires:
  level[cm]/1 -> 1-D Lookup Table/1, " "/1
  Switch/1 -> Scope1/1, Integrator/1
  Remote Heater/1 -> Switch/4
  TIC 705/1(Out1) -> Switch/2
  " "/1 -> Switch/1
  liter(dm^3)/1 -> m*c (mass*spesific heat of water)1/1
  "liter/s T-701 "/1 -> " Ketika level > 0 maka suhu dari T-701 sudah masuk ke tank F-705"/1, Integrator1/1
  Product4/1 -> Add2/2
  Add2/1 -> Divide3/1
  Product5/1 -> Add2/1
  dari Heat T-701/1 -> Product4/2
  Add3/1 -> Divide3/2
  1-D Lookup Table/1 -> Display2/1, Switch/3
  Thermocouple Transmitter (TT 705A)/1(Out2) -> TIC 705/2(In3)
  Set Point/1 -> Celcius to mA/1(In1)
  Celcius to mA/1(Out1) -> TIC 705/1(In2)
  Integrator/1 -> Product5/1, Display4/1
  Divide3/1 -> Thermocouple Transmitter (TT 705A)/1(In2), Display3/1, suhu/1
  Integrator1/1 -> m*c (mass*spesific heat of water)/1
  m*c (mass*spesific heat of water)1/1 -> Product5/2, Add3/1
  Product1/1 -> Add3/2
  m*c (mass*spesific heat of water)/1 -> Product1/2, Product4/3
  " Ketika level > 0 maka suhu dari T-701 sudah masuk ke tank F-705"/1 -> Product1/1, Product4/1

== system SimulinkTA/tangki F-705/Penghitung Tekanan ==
  Suhu : Inport  RequirementInfo={} %GIDa_58712087_af50_42a9_a9e9_5e3bcd7807c1
  Level : Inport  RequirementInfo={} %GIDa_22692da2_ddf7_4818_a8ae_ff05e98f017e  Port=2
  Bourdon Tube : Lookup_n-D  RequirementInfo={} %GIDa_e704bcb7_77b8_4090_ba97_d860dc590308  BreakpointsForDimension1=[28,29,30,31,32,33,34,35,36,37,38,39,40,41,42,43,44,45,46,47,48,49,50,51,52,53,54,55,56,57,58,59,60,61,62,63,64,65,66,67,68,69,70,71,72,73,74,75,76,77,78,79,80,81,82,83,84,85,86,87,88,89,90,91,92,93,94,95,96,97,98,99,100]  BreakpointsForDimension2=[20,30,40,50]  Table=reshape([0,0,0,0,0,0,0,0,0,0,0,0,0,0,0,0,0,0,0,0,0,0,0,0,0,0,0,0,0,0,0,0,0,0,0,0,0,0,0,0,0,0,0,0,0,0,0,0,0,0,0,0,1,6,7,8,10,10,11,11,12,13,14,15,15,16,18,19,20,20,21,24,25,0,0,0,0,0,0,0,0,0,0,0,0,0,0,0,0,0,0,0,0,0,0,0,0,0,0,0,0,0,0,0,0,0,0,0,0,0,0,0,0,0,0,0,0,0,0,0,0,1,4,9,10,10,11,12,13,14,14,15,15,16,18,19,20,21,23,25,25,25,26,28,29,30,0,0,0,0,0,0,0,0,0,0,0,0,0,0,0,0,0,0,0,0,0,0,0,0,0,0,0,0,0,0,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  InternalRulePriority=Speed  RndMeth=Simplest
  Display1 : Display
  To Workspace : ToWorkspace  VariableName=tekanan_gas  SampleTime=-1
  Pressure tangki (mbar) : Outport  RequirementInfo={} %GIDa_7d53dc43_d096_4c1f_bbc8_f2037a39fe0e
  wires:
  Suhu/1 -> Bourdon Tube/1
  Level/1 -> Bourdon Tube/2
  Bourdon Tube/1 -> To Workspace/1, Display1/1, Pressure tangki (mbar)/1

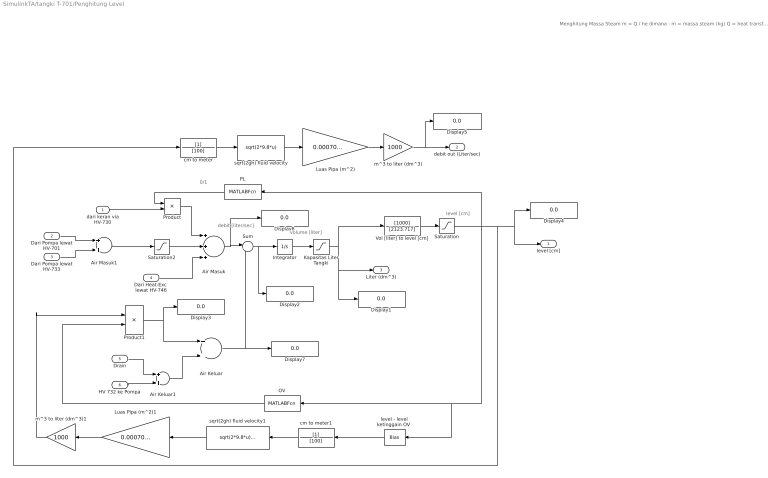
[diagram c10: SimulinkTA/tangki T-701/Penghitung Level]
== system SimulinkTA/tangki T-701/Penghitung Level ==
  note: 0/1
  note: debit [liter/sec]
  note: level [cm]
  note: volume [liter]
  note: Menghitung Massa Steam m = Q / he dimana : m = massa steam (kg) Q = heat transfer (J) he = Spesific laten heat evaporation (J/kg)
  dari keran via HV-730 : Inport  RequirementInfo={} %GIDa_f4a1d71d_0b7a_4bcc_9223_1d8a69ea52dc
  Dari Pompa lewat HV-701 : Inport  RequirementInfo={} %GIDa_bcd0222b_67c5_4ad0_ae15_9db113e7e14a  Port=2
  Dari Pompa lewat HV-733 : Inport  RequirementInfo={} %GIDa_4b8e73be_4259_45d7_b9cf_acd7ba1ec230  Port=3
  Dari Heat-Exc  lewat HV-746 : Inport  RequirementInfo={} %GIDa_f669825b_2b63_4428_a7ee_d7f2781b42ea  Port=4
  Drain : Inport  RequirementInfo={} %GIDa_05db6981_4386_4450_8fa6_87d3c7dae144  Port=5
  HV 732 ke Pompa : Inport  RequirementInfo={} %GIDa_4793ed22_7116_4518_85ec_5f7cc8139f75  Port=6
  Air Keluar : Sum  RequirementInfo={} %GIDa_3cd0728e_fe4b_414b_9e77_be6193ab9531
  Air Keluar1 : Sum  RequirementInfo={} %GIDa_bb354532_62ab_4772_a505_d82379f333d8
  Air Masuk : Sum  RequirementInfo={} %GIDa_cdd4ba05_cf24_489b_98bf_57e20333da77  Inputs=+++
  Air Masuk1 : Sum  RequirementInfo={} %GIDa_53e04d42_cb56_4b46_8247_c78245ebd565
  Display{1..5,7..8} (7 alike) : Display
  Integrator : Integrator  RequirementInfo={} %GIDa_1689616d_76ec_4ece_8d58_2618952534ef
  Kapasitas Liter Tangki : Saturate  RequirementInfo={} %GIDa_e5081ced_d9e7_4fa7_bb10_9d23d8b124cc  UpperLimit=120  LowerLimit=-99999999999999999999999999999999999999999999999999999999
  Luas Pipa (m^2) : Gain  RequirementInfo={} %GIDa_f5842acd_c41f_4ef0_a9fb_5b1efa83c212  Gain=0.000706858347
  Luas Pipa (m^2)1 : Gain  RequirementInfo={} %GIDa_7d37d097_3a80_4fb6_b115_617adc923876  Gain=0.000706858347
  OV : MATLABFcn  RequirementInfo={} %GIDa_3e19416b_9a04_48d8_8106_720a9a2232f8  MATLABFcn=OV
  PL : MATLABFcn  RequirementInfo={} %GIDa_2a9ae291_3bba_4f66_a1b0_1441e5ac2d96  MATLABFcn=PL
  Product : Product  RequirementInfo={} %GIDa_1308dd47_9330_4935_aaa7_a281df8f51dd
  Product1 : Product  RequirementInfo={} %GIDa_2188e6a4_80fd_4e5b_9655_ddbc3e33c6ec
  Saturation : Saturate  RequirementInfo={} %GIDa_79308d32_4d20_4b3b_a001_1757cf754c80  UpperLimit=65.5  LowerLimit=0
  Saturation2 : Saturate  RequirementInfo={} %GIDa_06a497b9_e1c0_4ffd_adcd_ae69bc4aaa1a  UpperLimit=1  LowerLimit=-999999999999999999999999999999999999999999999999999999
  Sum : Sum  RequirementInfo={} %GIDa_89d6290b_570a_4245_926b_4d36de9eadde  Inputs=|+-
  Vol [liter] to level [cm] : TransferFcn  RequirementInfo={} %GIDa_6cb2c5c2_16ba_4b47_aec7_7d5b41c36fa6  Numerator=[1000]  Denominator=[2123.717]
  cm to meter : TransferFcn  RequirementInfo={} %GIDa_8f6c046a_2359_4068_a8d9_6a7d70857493  Denominator=[100]
  cm to meter1 : TransferFcn  RequirementInfo={} %GIDa_74643c6a_4035_463e_bcea_ea5831f90c64  Denominator=[100]
  "level - level ketinggain OV " : Bias  RequirementInfo={} %GIDa_2ec32983_aa27_4878_aba5_49febe503e7f  Bias=-60
  m^3 to liter (dm^3) : Gain  RequirementInfo={} %GIDa_860744d2_a59e_4199_862e_1fc5d408b2ba  Gain=1000
  m^3 to liter (dm^3)1 : Gain  RequirementInfo={} %GIDa_2c7c523e_6a0c_4bbf_9386_ddb6376879d4  Gain=1000
  sqrt(2gh) fluid velocity : Fcn  RequirementInfo={} %GIDa_0f586cee_299a_4e56_b36a_90e41739e574  Expr=sqrt(2*9.8*u)
  sqrt(2gh) fluid velocity1 : Fcn  RequirementInfo={} %GIDa_dd97d7db_d9e9_430e_b572_9149a2d8c32b  Expr=sqrt(2*9.8*u)+0.00001
  level [cm] : Outport  RequirementInfo={} %GIDa_c62f379f_c1ba_4aea_bf08_0fcb69a7313e
  debit out (Liter/sec) : Outport  RequirementInfo={} %GIDa_ecadf756_1a47_4690_8dfd_3c05705f1405  Port=2
  Liter (dm^3) : Outport  RequirementInfo={} %GIDa_37f1eaa9_175a_409f_9397_d764201ba387  Port=3
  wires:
  Vol [liter] to level [cm]/1 -> Saturation/1
  Integrator/1 -> Kapasitas Liter Tangki/1
  Sum/1 -> Integrator/1, Display2/1
  Air Masuk/1 -> Display8/1, Sum/1
  Dari Heat-Exc  lewat HV-746/1 -> Air Masuk/3
  Product/1 -> Air Masuk/1
  dari keran via HV-730/1 -> Product/2
  PL/1 -> Product/1
  m^3 to liter (dm^3)1/1 -> Product1/1
  OV/1 -> Product1/2
  Product1/1 -> Display3/1, Air Keluar/1
  Drain/1 -> Air Keluar1/1
  HV 732 ke Pompa/1 -> Air Keluar1/2
  Air Keluar1/1 -> Air Keluar/2
  Air Keluar/1 -> Display7/1, Sum/2
  Saturation/1 -> "level - level ketinggain OV "/1, OV/1, level [cm]/1, Display4/1, cm to meter/1, PL/1
  m^3 to liter (dm^3)/1 -> Display5/1, debit out (Liter/sec)/1
  sqrt(2gh) fluid velocity/1 -> Luas Pipa (m^2)/1
  Luas Pipa (m^2)/1 -> m^3 to liter (dm^3)/1
  cm to meter/1 -> sqrt(2gh) fluid velocity/1
  cm to meter1/1 -> sqrt(2gh) fluid velocity1/1
  sqrt(2gh) fluid velocity1/1 -> Luas Pipa (m^2)1/1
  Luas Pipa (m^2)1/1 -> m^3 to liter (dm^3)1/1
  "level - level ketinggain OV "/1 -> cm to meter1/1
  Dari Pompa lewat HV-733/1 -> Air Masuk1/2
  Dari Pompa lewat HV-701/1 -> Air Masuk1/1
  Air Masuk1/1 -> Saturation2/1
  Saturation2/1 -> Air Masuk/2
  Kapasitas Liter Tangki/1 -> Vol [liter] to level [cm]/1, Display1/1, Liter (dm^3)/1

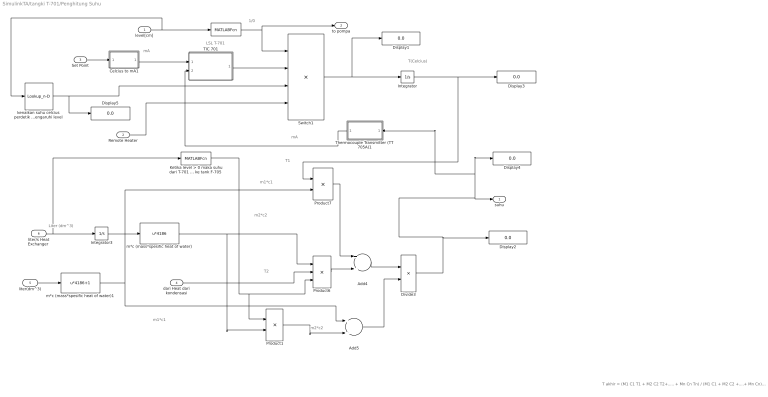
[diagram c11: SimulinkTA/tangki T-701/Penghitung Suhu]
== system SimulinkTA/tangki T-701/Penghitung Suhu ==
  note: mA
  note: mA
  note: T(Celcius)
  note: LSL T-701
  note: 1/0
  note: m1*c1
  note: T1
  note: m2*c2
  note: T2
  note: m2*c2
  note: m1*c1
  note: Liter (dm^3)
  note: T akhir = (M1 C1 T1 + M2 C2 T2+..... + Mn Cn Tn) / (M1 C1 + M2 C2 +....+ Mn Cn) dimana : T akhir = final temperatur M = massa air C = spesific heat (Kj/Kg C ) T1..n = temperatur subtansi
  level[cm] : Inport  RequirementInfo={} %GIDa_d5c686e8_6085_4a32_891e_69ed11b6461b
  Remote Heater : Inport  RequirementInfo={} %GIDa_4bb99a57_bcae_4944_8bac_257577f9ee2f  Port=2
  Set Point : Inport  RequirementInfo={} %GIDa_cbc18549_bce2_4b90_b762_270ad8569e82  Port=3
  dari Heat dari kondensasi : Inport  RequirementInfo={} %GIDa_6dc053b8_1154_47a7_8195_702e320e1195  Port=4
  liter(dm^3) : Inport  RequirementInfo={} %GIDa_a05cc77c_9e92_4b88_8277_c84ca0d8f024  Port=5
  "liter/s Heat Exchanger " : Inport  RequirementInfo={} %GIDa_1a7e391b_04ad_41e6_bb89_61de82d2f779  Port=6
  " " : MATLABFcn  RequirementInfo="{'linktype_rmi_simulink' 'D' ':376' 'true' 'D/Lamp  (SubSystem)' '' } %GIDa_dca3b9da_3842_4c8b_8255_19f997a60c38"  MATLABFcn=LSL
  " Ketika level > 0 maka suhu dari T-701 sudah masuk ke tank F-705" : MATLABFcn  RequirementInfo={} %GIDa_847c8835_2721_47ad_af63_e3c188af7392  MATLABFcn=HeatF705
  Add4 : Sum  RequirementInfo={} %GIDa_776d31fd_ce8e_48e5_bfe4_5bea15b697c7
  Add5 : Sum  RequirementInfo={} %GIDa_307d5198_2c0b_4d04_9cc2_1331a41dab9e
  Celcius to mA1 : Subsystem  RequirementInfo={} %GIDa_852a575d_74bb_486c_93bd_04e6c7b6ee85
  Display{1..5} (5 alike) : Display
  Divide3 : Product  RequirementInfo={} %GIDa_7452abf4_a473_4671_861f_b492ca17cf9b  Inputs=*/
  Integrator : Integrator  RequirementInfo={} %GIDa_9c3a9a48_5811_4736_a57a_6b2b05970242  InitialCondition=31.5
  Integrator3 : Integrator  RequirementInfo={} %GIDa_e4c8ff84_3631_4c9d_9393_e7783a05625a
  Product1 : Product  RequirementInfo={} %GIDa_02ddb7c1_4053_4c7f_850d_df8e58ded710
  Product6 : Product  RequirementInfo={} %GIDa_3da60934_517f_4c16_8bd8_6b5b7a8012cd  Inputs=3
  Product7 : Product  RequirementInfo={} %GIDa_8ca998fb_d629_4a2f_8ffb_d22c01684fd0
  Switch1 : Product  RequirementInfo={} %GIDa_b7105f57_0a4a_4bcc_80e0_294f1051dbfb  Inputs=4
  TIC 701 : Subsystem  RequirementInfo={} %GIDa_5c9139c2_7f6b_4ce1_87c4_711e11143567
  Thermocouple Transmitter (TT 705A)1 : Subsystem  RequirementInfo={} %GIDa_653a71cf_0970_46c4_9d09_e29f33daed12
  kenaikan suhu celcius perdetik yang dipengaruhi level : Lookup_n-D  NumberOfTableDimensions=1  BreakpointsForDimension1=[20,30,40,50]  Table=[0.093322,0.0671,0.0528,0.04138]  InternalRulePriority=Speed  RndMeth=Simplest
  m*c (mass*spesific heat of water) : Fcn  RequirementInfo={} %GIDa_076221fe_9f79_4248_bbc1_ed2db8f2abf2  Expr=u*4186
  m*c (mass*spesific heat of water)1 : Fcn  RequirementInfo={} %GIDa_2e425061_0f2a_41ad_aa92_ad387bde30fe  Expr=u*4186+1
  suhu : Outport  RequirementInfo={} %GIDa_5365b8a2_25b8_482a_8405_0315cb80f8b9
  to pompa : Outport  RequirementInfo={} %GIDa_4653359b_31f7_45f7_b677_0756898094ae  Port=2
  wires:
  Switch1/1 -> Display1/1, Integrator/1
  Remote Heater/1 -> Switch1/4
  TIC 701/1(Out1) -> Switch1/2
  " "/1 -> Switch1/1, to pompa/1
  liter(dm^3)/1 -> m*c (mass*spesific heat of water)1/1
  "liter/s Heat Exchanger "/1 -> " Ketika level > 0 maka suhu dari T-701 sudah masuk ke tank F-705"/1, Integrator3/1
  Product6/1 -> Add4/2
  Add4/1 -> Divide3/1
  Product7/1 -> Add4/1
  dari Heat dari kondensasi/1 -> Product6/2
  Add5/1 -> Divide3/2
  Integrator3/1 -> m*c (mass*spesific heat of water)/1
  kenaikan suhu celcius perdetik yang dipengaruhi level/1 -> Display5/1, Switch1/3
  Thermocouple Transmitter (TT 705A)1/1(Out1) -> TIC 701/2(In2)
  Set Point/1 -> Celcius to mA1/1(In1)
  Celcius to mA1/1(Out1) -> TIC 701/1(In1)
  m*c (mass*spesific heat of water)1/1 -> Add5/1, Product7/2
  Divide3/1 -> suhu/1, Thermocouple Transmitter (TT 705A)1/1(In1), Display4/1, Display2/1
  Integrator/1 -> Display3/1, Product7/1
  m*c (mass*spesific heat of water)/1 -> Product1/2, Product6/1
  " Ketika level > 0 maka suhu dari T-701 sudah masuk ke tank F-705"/1 -> Product1/1, Product6/3
  Product1/1 -> Add5/2
  level[cm]/1 -> kenaikan suhu celcius perdetik yang dipengaruhi level/1, " "/1

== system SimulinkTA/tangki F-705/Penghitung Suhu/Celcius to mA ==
  In1 : Inport  RequirementInfo={} %GIDa_fbf10dfa_1813_4050_9a5b_3efe7b854fa1
  Add : Sum  RequirementInfo={} %GIDa_be9b0146_a83c_4e8b_9cce_649d0bdc96a4
  initial condition (mA) : Constant  RequirementInfo={} %GIDa_6dcc9700_f7db_4f5d_8426_c2d95f91fa63  Value=4
  to mA : Gain  RequirementInfo={} %GIDa_1c4531d4_5c53_45ea_9dbf_710e25517081  Gain=0.16
  Out1 : Outport  RequirementInfo={} %GIDa_9112969c_0bdb_44ef_bd93_4169d92d4508
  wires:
  In1/1 -> to mA/1
  to mA/1 -> Add/1
  Add/1 -> Out1/1
  initial condition (mA)/1 -> Add/2

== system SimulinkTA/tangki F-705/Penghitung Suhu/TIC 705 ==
  note: 1/0
  In2 : Inport  RequirementInfo={} %GIDa_c15110f2_cfe8_40d8_90e5_90373ba12970
  In3 : Inport  RequirementInfo={} %GIDa_95ef785b_97cd_43e8_90ed_0a50fccd3b87  Port=2
  ON/OFF Controller : MATLABFcn  RequirementInfo={} %GIDa_f81e3f88_ddce_4853_80c2_cbdb29acc973  MATLABFcn=TM
  Sum1 : Sum  RequirementInfo={} %GIDa_204986ff_1bce_4b4c_acac_834d20687a0d  Inputs=|+-
  Out1 : Outport  RequirementInfo={} %GIDa_be5608b1_3e37_4d52_a584_c784d913480c
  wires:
  In3/1 -> Sum1/2
  Sum1/1 -> ON/OFF Controller/1
  In2/1 -> Sum1/1
  ON/OFF Controller/1 -> Out1/1

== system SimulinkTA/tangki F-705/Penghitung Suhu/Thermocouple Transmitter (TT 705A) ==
  In2 : Inport  RequirementInfo={} %GIDa_085c313f_6fae_4a08_9c8a_243ad7344bb8
  Bias : Bias  RequirementInfo={} %GIDa_45411e6c_eb1c_488d_9e12_40acc474404d  Bias=4
  Thermocouple Sensor : TransferFcn  RequirementInfo={} %GIDa_34c19b0a_cf8d_43b0_9768_dc52c83c4b4d  Numerator=[0.16]  Denominator=[1 1]
  Out2 : Outport  RequirementInfo={} %GIDa_5aae600f_3a36_4ffa_b87f_93ea464abb9e
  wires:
  Bias/1 -> Out2/1
  In2/1 -> Thermocouple Sensor/1
  Thermocouple Sensor/1 -> Bias/1

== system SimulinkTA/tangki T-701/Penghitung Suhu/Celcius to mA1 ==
  In1 : Inport  RequirementInfo={} %GIDa_c76dcbc9_ba75_48b6_a7a7_a83a1745e5fa
  Add : Sum  RequirementInfo={} %GIDa_bdc5a29a_1709_4d55_99cd_17c4e5df383d
  initial condition (mA) : Constant  RequirementInfo={} %GIDa_2cedaf6d_ccba_4766_a6a3_d346a062cf08  Value=4
  to mA : Gain  RequirementInfo={} %GIDa_147c7531_76b7_41a0_be76_a1ba5f72c698  Gain=0.16
  Out1 : Outport  RequirementInfo={} %GIDa_47c1abb4_7120_4db9_8a97_2231a5a099d5
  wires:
  In1/1 -> to mA/1
  to mA/1 -> Add/1
  Add/1 -> Out1/1
  initial condition (mA)/1 -> Add/2

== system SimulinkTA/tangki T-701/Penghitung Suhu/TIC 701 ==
  note: 1/0
  In1 : Inport  RequirementInfo={} %GIDa_80cfac6e_66f1_43f2_8c0d_e5a61631cddd
  In2 : Inport  RequirementInfo={} %GIDa_67f053ff_f2f3_4587_be3c_c5d2f84602f8  Port=2
  ON/OFF Controller : MATLABFcn  RequirementInfo={} %GIDa_b883d62c_d34b_40d1_aa89_76863ace6a38  MATLABFcn=TM
  Sum1 : Sum  RequirementInfo={} %GIDa_587ff269_8a95_4ff2_a85b_fcdb1d0e6f39  Inputs=|+-
  Out1 : Outport  RequirementInfo={} %GIDa_7e1bbe53_f268_49c8_8e7b_af2244337b8e
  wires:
  In2/1 -> Sum1/2
  Sum1/1 -> ON/OFF Controller/1
  In1/1 -> Sum1/1
  ON/OFF Controller/1 -> Out1/1
